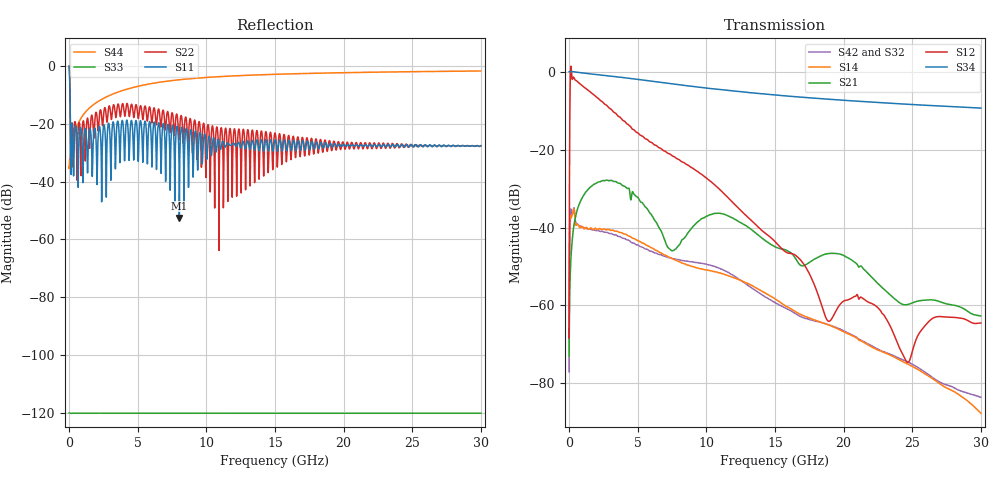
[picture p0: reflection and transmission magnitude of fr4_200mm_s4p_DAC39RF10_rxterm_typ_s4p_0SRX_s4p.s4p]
! Touchstone generated by fitter/viewer
# HZ S  RI R 5.000000e+01
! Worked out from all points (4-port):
!   3599 points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, 8.336 MHz to 30 GHz, reference 50 ohm
!   strongest paths, dB at 8.336 MHz, 7.502 GHz, 15 GHz, 22.51 GHz, 30 GHz:
!     S34: 0.2, -2.9, -5.8, -7.8, -9.2
!     S12: -68.4, -21.5, -43.6, -60.6, -64.5
!     S21: -73.1, -45.9, -44.9, -54.4, -62.7
!     S14: -71.2, -47.9, -58.3, -71.5, -87.8
!     S42: -77.1, -47.9, -59.3, -71.3, -83.7
!     S32: -77.1, -47.9, -59.3, -71.3, -83.7
!   lowest |S11| = -52.5 dB at 8.036 GHz (marker M1), VSWR 1.00, Z = 50 + j0.233 ohm
!   |S11| at or under -10 dB: 74 MHz to end of sweep
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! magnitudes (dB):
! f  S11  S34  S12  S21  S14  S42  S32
! 8.336 MHz  -0.1  0.2  -68.4  -73.1  -71.2  -77.1  -77.1
! 233.4 MHz  -20.2  0.2  -1.8  -43.3  -36.7  -36.6  -36.6
! 2.776 GHz  -25.4  -0.9  -8.6  -27.7  -40.5  -41.2  -41.2
! 8.036 GHz  -52.5  -3.2  -22.5  -44.4  -48.7  -48.2  -48.2
! 18.88 GHz  -28.2  -6.9  -64.0  -46.6  -65.0  -64.9  -64.9
! 24.67 GHz  -27.4  -8.2  -74.7  -59.8  -75.1  -74.5  -74.5
! 30 GHz  -27.6  -9.2  -64.5  -62.7  -87.8  -83.7  -83.7
